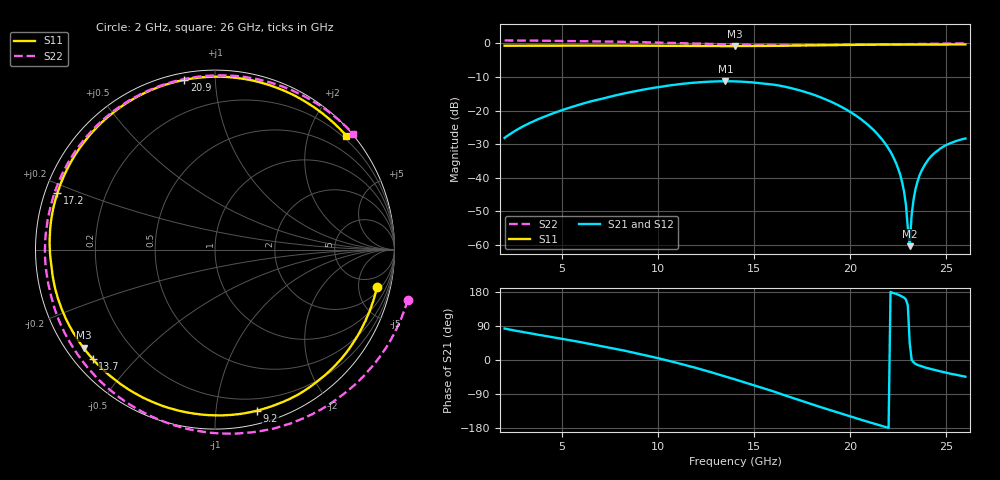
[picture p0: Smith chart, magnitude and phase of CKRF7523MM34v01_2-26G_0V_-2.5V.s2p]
! CHUO DENSHI KOGYO Co.,Ltd.
! 8. May 2017
! CKRF7523MM34_RT5880
! N-channel HJ-FET
! Vds = 0V Vgs = -2.5V
# Hz S  MA  R 50
!	f	S11	S21	S12	S22
!	Hz	MAG	ANG	MAG	ANG	MAG	ANG	MAG	ANG
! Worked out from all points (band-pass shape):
!   241 points, 2 GHz to 26 GHz, reference 50 ohm
!   highest |S21| = -11.26 dB at 13.5 GHz (marker M1); lowest = -60.4 dB at 23.1 GHz (marker M2)
!   |S21| within 3 dB of the highest: 8.763 GHz to 17.54 GHz (8.78 GHz wide, 66.8 % of centre)
!   lowest |S11| = -0.8 dB at 14 GHz (marker M3), VSWR 22.29, Z = 2.49 - j16.6 ohm
!   |S11| at or under -10 dB: nowhere
!   |S22| runs from -0.5 to 0.9 dB; largest |S21 - S12| = 0.00037
!   S11 on the Smith chart (normalised r, x): 2 GHz: 2.70, -7.92; 9.2 GHz: 0.10, -1.29; 13.7 GHz: 0.05, -0.38; 17.2 GHz: 0.04, +0.17; 20.9 GHz: 0.03, +0.83; 26 GHz: 0.13, +2.67
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2e9  0.9266 -12.9  0.03913 83.1  0.03926 83.2  1.11 -14.6
6e9  0.9297 -43.9  0.1251 46.7  0.1252 46.6  1.084 -44.1
9.2e9  0.9277 -75.3  0.2045 14.1  0.2045 14.1  1.043 -75.1
1e10  0.9254 -84.7  0.2238 4.7  0.2237 4.7  1.03 -84.1
1.18e10  0.9187 -108.6  0.2593 -18.6  0.2594 -18.7  0.9999 -106.5
1.35e10  0.9141 -134.9  0.2734 -43.4  0.2734 -43.5  0.9736 -130.0
1.37e10  0.9141 -138.2  0.2731 -46.5  0.2732 -46.5  0.9711 -133.0
1.4e10  0.9141 -143.3  0.2721 -51.2  0.2721 -51.1  0.967 -137.4
1.56e10  0.9162 -171.3  0.2501 -76.3  0.2499 -76.2  0.9503 -162.2
1.72e10  0.9328 160.3  0.2062 -103.4  0.2062 -103.5  0.9465 171.8
1.8e10  0.941 146.3  0.176 -116.8  0.1761 -116.8  0.9488 158.4
1.95e10  0.9537 121.4  0.1152 -141.1  0.1153 -141.2  0.9546 133.1
2.09e10  0.9612 100.2  0.06212 -162.8  0.06205 -162.9  0.9618 110.0
2.2e10  0.9642 85.2  0.02703 -179.2  0.02712 -179.3  0.9695 92.8
2.27e10  0.9651 76.3  0.00864 167.5  0.00873 168.4  0.9749 82.3
2.29e10  0.9651 73.9  0.00402 159.9  0.00398 158.7  0.9765 79.4
2.31e10  0.9652 71.5  0.00095 44.9  0.00087 40.2  0.9779 76.5
2.32e10  0.9651 70.3  0.00278 0.7  0.00271 -3.3  0.9788 75.1
2.33e10  0.9652 69.1  0.0047 -5.8  0.00468 -7.4  0.9795 73.7
2.37e10  0.9656 64.5  0.01238 -16.2  0.01247 -16.2  0.9829 68.2
2.46e10  0.9663 54.8  0.02591 -28.7  0.02604 -28.8  0.991 56.4
2.6e10  0.9679 40.9  0.03824 -44.0  0.03834 -44.3  1.004 39.9
